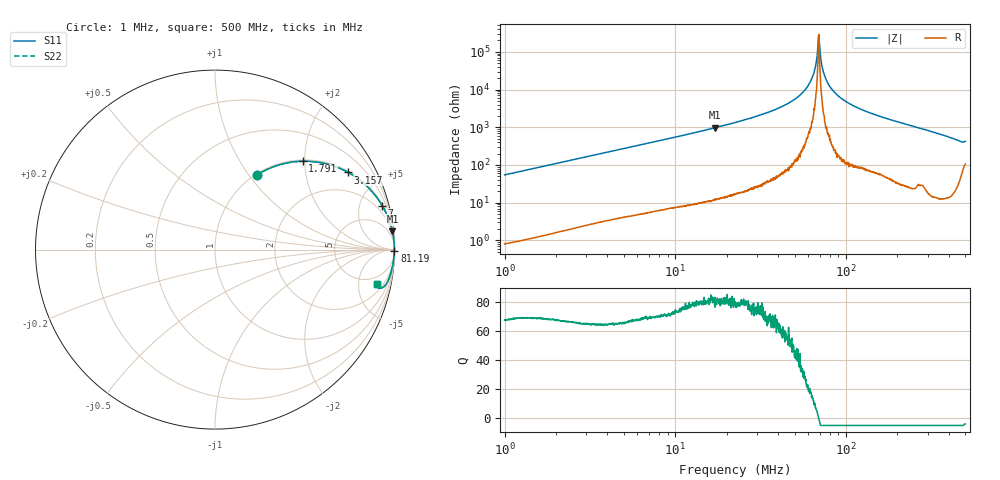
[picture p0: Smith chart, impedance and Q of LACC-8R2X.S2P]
!s-Parameter Generated by FASTRON Sdn. Bhd.
!FASTRON P/N : LACC-8R2X
!Keysight Technologies,E4991B,MY54100416,A.01.15
!Date: Wed Mar 18 09:23:59 2026
!Version  : Rev00 Wed Mar 18 09:23:59 2026
!Data & Calibration Information:
!PortZ  Port1:50+j0  Port2:50+j0
!When reading, reference impedance value at option line is always used.
!Remarks : This data is being provided solely for informational purposes.
!Freq	S11	S21	S12	S22
# Hz S dB R 50
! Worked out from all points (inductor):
!   1601 points, 1 MHz to 500 MHz, reference 50 ohm
!   read as one part in series: L = 8.68 uH near 1.032 MHz
!   highest Q = 82.4 at 17.1 MHz (marker M1), where L = 9.03 uH
!   self-resonance near 68.97 MHz
!   S11 on the Smith chart (normalised r, x): 1 MHz: 1.02, +1.09; 1.791 MHz: 1.03, +1.95; 3.157 MHz: 1.05, +3.42; 7 MHz: 1.11, +7.59; 81.19 MHz: open; 500 MHz: 3.10, -8.29
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1000000  -6.44 60.7  -1.19 -28.4  -1.19 -28.4  -6.44 60.7
1790723  -3.18 45.3  -2.96 -43.9  -2.96 -43.9  -3.18 45.3
2820919  -1.60 32.9  -5.30 -56.2  -5.30 -56.2  -1.60 32.9
3157253  -1.33 30.1  -6.00 -59.1  -6.00 -59.1  -1.33 30.1
7000273  -0.32 14.7  -11.91 -74.5  -11.91 -74.5  -0.32 14.7
7957584  -0.25 13.0  -12.96 -76.2  -12.96 -76.2  -0.25 13.0
1.710377e7  -0.06 5.9  -19.80 -83.4  -19.80 -83.4  -0.06 5.9
2.236068e7  -0.03 4.3  -22.50 -85.0  -22.50 -85.0  -0.03 4.3
4.641026e7  -0.01 1.3  -32.97 -87.7  -32.97 -87.7  -0.01 1.3
5.613968e7  -0.00 0.7  -38.72 -87.4  -38.72 -87.4  -0.00 0.7
6.307767e7  -0.00 0.3  -45.87 -85.7  -45.87 -85.7  -0.00 0.3
6.557589e7  -0.00 0.2  -50.51 -83.4  -50.51 -83.4  -0.00 0.2
6.790877e7  -0.00 0.1  -59.23 -74.5  -59.23 -74.5  -0.00 0.1
6.950996e7  -0.00 -0.0  -67.90 41.0  -67.90 41.0  -0.00 -0.0
7.059833e7  -0.00 -0.1  -58.80 75.8  -58.80 75.8  -0.00 -0.1
7.254416e7  -0.00 -0.1  -51.67 83.6  -51.67 83.6  -0.00 -0.1
7.425464e7  -0.00 -0.2  -48.15 85.3  -48.15 85.3  -0.00 -0.2
8.11935e7  -0.00 -0.5  -41.02 87.3  -41.02 87.3  -0.00 -0.5
9.122775e7  -0.00 -0.9  -36.16 87.6  -36.16 87.6  -0.00 -0.9
1.069764e8  -0.01 -1.4  -32.04 87.2  -32.04 87.2  -0.01 -1.4
1.77937e8  -0.03 -3.5  -24.31 85.0  -24.31 85.0  -0.03 -3.5
5e8  -0.68 -12.1  -13.30 63.7  -13.30 63.7  -0.68 -12.1
